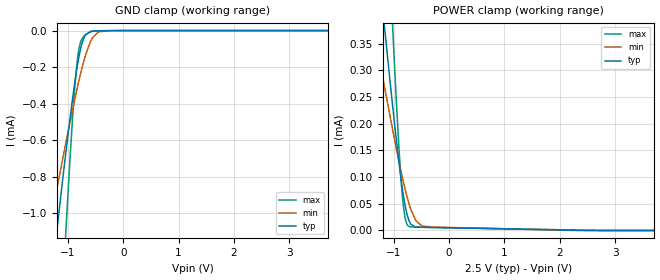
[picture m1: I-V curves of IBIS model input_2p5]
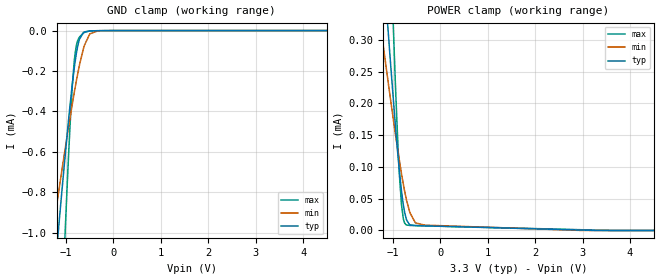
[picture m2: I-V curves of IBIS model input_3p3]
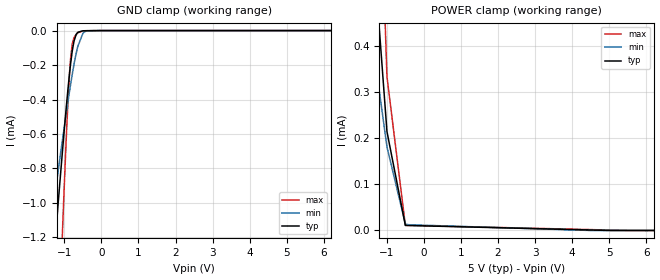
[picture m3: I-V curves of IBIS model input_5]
|Texas Instruments Incorporated
|Low-Noise 1A Transformer Driver for Isolated Power Supplies,Internal
|Clock-150kHz
| Marketing part#   Digital Voltage Range   Package-type   #pins
| SN6505BDBVR   2.25V-5.5V   SOT23   6
| SN6505BDBVT   2.25V-5.5V   SOT23   6
[IBIS Ver]   4.1
[File name]   sn6505b.ibs
[File Rev]   1.0
[Date]   10/6/2015
[Source]
| Texas Instruments Incorporated.
| Analog-eLab Design Center, HPA
| 12500 TI Blvd
| Dallas, TX -75243
[Notes]   Revision History:
| Rev 1.0: 10/6/2015
| - Initial version of the model
| - Model generated from simulations in TISPICE
| - Model matched to SPICE simulation
| - C_comp although listed in numerical order of value are
|   obtained from varying PVT conditions. For PVT conditions for
|   each specific value refer the buffer description under
|   respective [Model]. IBIS model user is responsible for using
|   appropriate C_comp to simulate for Signal Integrity.
|*EXCEPTION:   *
|* There are leakage currents in Power Clamp IV table becasue of a Pulldown *
|* resistor (R0) is connected to Pad.   *
[Disclaimer]
| This model is designed as an aid for customers of Texas Instruments.
| TI and its licensors and suppliers make no warranties, either expressed
| or implied, with respect to this  model, including the warranties of
| merchantability or fitness for a particular purpose. The model is
| provided solely on an "as is" basis. The entire risk as to its quality
| and performance is with the customer.
[Copyright]
(C) Copyright 2015 Texas Instruments Incorporated.All rights reserved.
|   SN6505BDBV
[Component]   SN6505BDBV
[Manufacturer]   TI
[Package]   |6 SOT23 - DBV package
|   typ   min   max
R_pkg   0.1   0.08   0.12
L_pkg   1.0nH   0.8nH   1.2nH
C_pkg   0.2pF   0.16pF   0.24pF
[Pin]  signal_name   model_name   R_pin   L_pin   C_pin
1   D1   NC   NA   NA   NA
2   VCC   POWER   NA   NA   NA
3   D2   NC   NA   NA   NA
4   GND   GND   NA   NA   NA
5   EN   INPUT   NA   NA   NA
6   CLK   INPUT   NA   NA   NA
|   Model Selectors
[Model Selector] INPUT
input_2p5   2.5V  digital Input
input_3p3   3.3V  digital Input
input_5   5.0V  digital Input
| Models and submodels in the file (3): input_2p5 (Input), input_3p3 (Input), input_5 (Input)
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|   input_2p5 Model
[Model]   input_2p5
Model_type   Input
Vinl = 0.75
Vinh = 1.75
|   typ   min   max
|   (nom PVT)   (fast PVT)   (slow PVT)
C_comp   6.624e-13   5.025e-13   8.075e-13
[Model spec]
|subparameter
Vinl   0.75   0.675   0.825
Vinh   1.75   1.575   1.925
| Where nom  PVT is Nominal Process, 2.5V, 27C
|   Fast PVT is Strong Process,  2.75V, -40C
|   Slow PVT is Weak Process,   2.25V, 150C
[Voltage Range]   2.5   2.25   2.75
|Junction Temperature
[Temperature Range]   27   150   -40
[Power Clamp Reference]   2.5   2.25   2.75
[GND Clamp Reference]   0   0   0
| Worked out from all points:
|   GND clamp passes 1 mA (typ) near -1.16 V on its own axis
[GND Clamp]
|   Voltage   I(typ)   I(min)   I(max)
-2.5V     -4.742mA   -3.013mA   -10.16mA
-1.367V   -1.546mA   -1.135mA   -3.031mA
-1.224V   -1.157mA   -905.8uA   -2.17mA
-1.042V   -678.4uA   -621.4uA   -1.122mA
-910.5mV  -359.3uA   -425.1uA   -450.3uA
-832.7mV  -197.2uA   -315.8uA   -167uA
-757.5mV  -81.93uA   -218.4uA   -52.11uA
-685mV    -24.63uA   -137.2uA   -23.15uA
-591.5mV  -4.784uA   -58.85uA   -6.676uA
-450.2mV  -1.041uA   -7uA       -1.026uA
-250mV    -500.7nA   -680.5nA   -466.3nA
5V        0A         0A         0A
[POWER Clamp]
|   Voltage   I(typ)   I(min)   I(max)
-2.5V     1.82mA     1.049mA    3.909mA
-1.355V   576.5uA    374.7uA    1.144mA
-1.188V   402.1uA    280.5uA    755.6uA
-1.053V   265.2uA    206.1uA    451.2uA
-976.5mV  190.9uA    165.3uA    288uA
-905mV    126.2uA    128.7uA    151.7uA
-841.7mV  76.04uA    98.16uA    61.23uA
-784mV    40.85uA    72.68uA    18.5uA
-711.3mV  15.06uA    45.62uA    7.003uA
-592mV    6.36uA     17.35uA    6.234uA
-486.3mV  5.978uA    8.166uA    6.035uA
5V        0A         0A         0A
|   input_3p3 Model
[Model]   input_3p3
Model_type   Input
Vinl = 0.99
Vinh = 2.31
|   typ   min   max
|   (nom PVT)   (fast PVT)   (slow PVT)
C_comp   6.233e-13   4.754e-13   7.578e-13
[Model spec]
|subparameter
Vinl   0.99   0.90   1.08
Vinh   2.31   2.10   2.52
| Where nom  PVT is Nominal Process, 3.3V, 27C
|   Fast PVT is Strong Process,  3.6V, -40C
|   Slow PVT is Weak Process,   3V, 150C
[Voltage Range]   3.3   3   3.6
|Junction Temperature
[Temperature Range]   27   150   -40
[Power Clamp Reference]   3.3   3   3.6
[GND Clamp Reference]   0   0   0
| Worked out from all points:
|   GND clamp passes 1 mA (typ) near -1.16 V on its own axis
|   POWER clamp passes 1 mA (typ) near -1.75 V on its own axis
[GND Clamp]
|   Voltage   I(typ)   I(min)   I(max)
-3.3V     -7.037mA   -4.364mA   -15.27mA
-1.406V   -1.654mA   -1.199mA   -3.271mA
-1.257V   -1.246mA   -958.3uA   -2.366mA
-1.216V   -1.134mA   -892.5uA   -2.12mA
-1.063V   -731.1uA   -653uA     -1.237mA
-974.4mV  -509.8uA   -519.2uA   -760.5uA
-874.5mV  -280.4uA   -373.6uA   -301.1uA
-815.1mV  -165.6uA   -292uA     -126uA
-716.1mV  -42.77uA   -170.2uA   -32.28uA
-610.5mV  -6.544uA   -72.02uA   -8.933uA
-327mV    -659nA     -1.143uA   -612.7nA
6.6V      0A         0A         0A
[POWER Clamp]
|   Voltage   I(typ)   I(min)   I(max)
-3.3V     2.704mA    1.531mA    5.867mA
-1.242V   459.5uA    312.5uA    881.5uA
-1.182V   397.3uA    278.9uA    742.8uA
-1.049V   263uA      205.9uA    444.4uA
-952.8mV  170.4uA    154.8uA    242uA
-871.2mV  99.83uA    114uA      99.86uA
-819.6mV  62.68uA    89.95uA    41.78uA
-774mV    37.68uA    70.47uA    16.49uA
-718.8mV  18.4uA     49.99uA    8.831uA
-525mV    7.668uA    11.93uA    7.692uA
-330mV    7.263uA    8.418uA    7.328uA
6.6V      0A         0A         0A
|   input_5 Model
[Model]   input_5
Model_type   Input
Vinl = 1.5
Vinh = 3.5
|   typ   min   max
|   (nom PVT)   (fast PVT)   (slow PVT)
C_comp   5.686e-13   4.317e-13   6.880e-13
[Model spec]
|subparameter
Vinl   1.5   1.35   1.65
Vinh   3.5   3.15   3.85
| Where nom  PVT is Nominal Process, 5V, 27C
|   Fast PVT is Strong Process,  5.5V, -40C
|   Slow PVT is Weak Process,   4.5V, 150C
[Voltage Range]   5   4.5   5.5
|Junction Temperature
[Temperature Range]   27   150   -40
[Power Clamp Reference]   5   4.5   5.5
[GND Clamp Reference]   0   0   0
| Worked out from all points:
|   GND clamp passes 1 mA (typ) near -1.17 V on its own axis
[GND Clamp]
|   Voltage   I(typ)   I(min)   I(max)
-5V       -11.95mA   -7.257mA   -26.2mA
-1.571V   -2.111mA   -1.467mA   -4.287mA
-1.337V   -1.464mA   -1.087mA   -2.848mA
-1.15V    -959.4uA   -788.9uA   -1.735mA
-1.04V    -673.4uA   -618.4uA   -1.111mA
-927.5mV  -398.2uA   -449.8uA   -528.4uA
-833mV    -197.7uA   -316.1uA   -167.7uA
-781.5mV  -112.9uA   -248.3uA   -73.36uA
-635mV    -9.988uA   -91.15uA   -12.65uA
-500mV    -1.474uA   -16.81uA   -1.662uA
-336mV    -678.4nA   -1.244uA   -630.6nA
10V       0A         0A         0A
[POWER Clamp]
|   Voltage   I(typ)   I(min)   I(max)
-5V       185.6mA    66.88mA    302.3mA
-3.321V   2.732mA    1.547mA    5.929mA
-996mV    214.4uA    181.2uA    333.5uA
-500mV    11.01uA    14.36uA    11.19uA
-310mV    10.62uA    12.14uA    10.83uA
4.5V      1.001uA    0A         1.866uA
5.5V      0A         0A         0A
10V       0A         0A         0A
